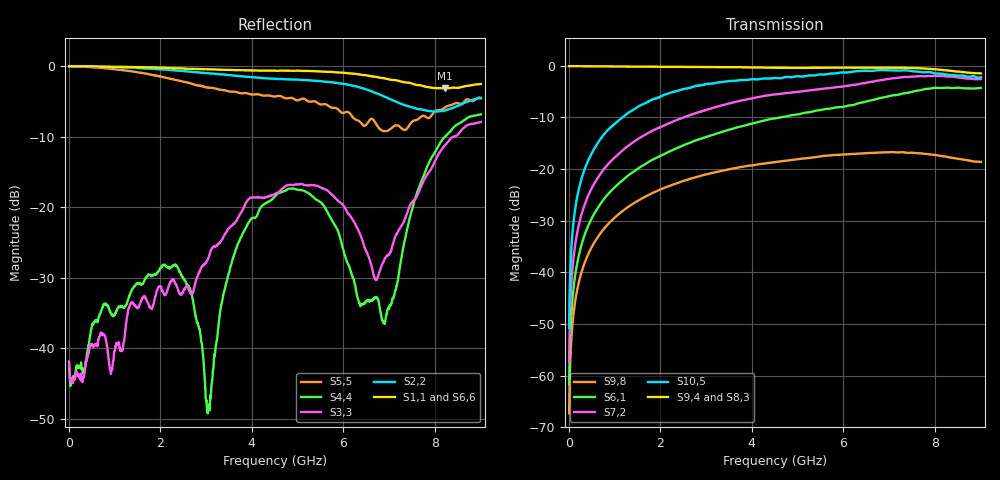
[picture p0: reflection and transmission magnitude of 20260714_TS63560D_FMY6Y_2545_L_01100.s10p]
# GHz S DB R 50
! CMT, SN0916, 25263762, 26.7.0
! Date: 15.07.2026 13:39:32
! Data: Format
! Freq S1.1:dB/Ang S1.2:dB/Ang S1.3:dB/Ang S1.4:dB/Ang S1.5:dB/Ang S1.6:dB/Ang S1.7:dB/Ang S1.8:dB/Ang S1.9:dB/Ang S1.10:dB/Ang
!  S2.1:dB/Ang S2.2:dB/Ang S2.3:dB/Ang S2.4:dB/Ang S2.5:dB/Ang S2.6:dB/Ang S2.7:dB/Ang S2.8:dB/Ang S2.9:dB/Ang S2.10:dB/Ang
!  S3.1:dB/Ang S3.2:dB/Ang S3.3:dB/Ang S3.4:dB/Ang S3.5:dB/Ang S3.6:dB/Ang S3.7:dB/Ang S3.8:dB/Ang S3.9:dB/Ang S3.10:dB/Ang
!  S4.1:dB/Ang S4.2:dB/Ang S4.3:dB/Ang S4.4:dB/Ang S4.5:dB/Ang S4.6:dB/Ang S4.7:dB/Ang S4.8:dB/Ang S4.9:dB/Ang S4.10:dB/Ang
!  S5.1:dB/Ang S5.2:dB/Ang S5.3:dB/Ang S5.4:dB/Ang S5.5:dB/Ang S5.6:dB/Ang S5.7:dB/Ang S5.8:dB/Ang S5.9:dB/Ang S5.10:dB/Ang
!  S6.1:dB/Ang S6.2:dB/Ang S6.3:dB/Ang S6.4:dB/Ang S6.5:dB/Ang S6.6:dB/Ang S6.7:dB/Ang S6.8:dB/Ang S6.9:dB/Ang S6.10:dB/Ang
!  S7.1:dB/Ang S7.2:dB/Ang S7.3:dB/Ang S7.4:dB/Ang S7.5:dB/Ang S7.6:dB/Ang S7.7:dB/Ang S7.8:dB/Ang S7.9:dB/Ang S7.10:dB/Ang
!  S8.1:dB/Ang S8.2:dB/Ang S8.3:dB/Ang S8.4:dB/Ang S8.5:dB/Ang S8.6:dB/Ang S8.7:dB/Ang S8.8:dB/Ang S8.9:dB/Ang S8.10:dB/Ang
!  S9.1:dB/Ang S9.2:dB/Ang S9.3:dB/Ang S9.4:dB/Ang S9.5:dB/Ang S9.6:dB/Ang S9.7:dB/Ang S9.8:dB/Ang S9.9:dB/Ang S9.10:dB/Ang
!  S10.1:dB/Ang S10.2:dB/Ang S10.3:dB/Ang S10.4:dB/Ang S10.5:dB/Ang S10.6:dB/Ang S10.7:dB/Ang S10.8:dB/Ang S10.9:dB/Ang S10.10:dB/Ang
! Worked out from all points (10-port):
!   2001 points, 10 MHz to 9 GHz, reference 50 ohm
!   strongest paths, dB at 10 MHz, 2.257 GHz, 4.505 GHz, 6.753 GHz, 9 GHz:
!     S9,4: -0.1, -0.2, -0.4, -0.4, -1.5
!     S8,3: -0.1, -0.2, -0.4, -0.4, -1.3
!     S10,5: -50.8, -5.1, -2.4, -0.8, -2.2
!     S7,2: -57.4, -10.9, -5.6, -2.9, -2.6
!     S6,1: -61.7, -16.4, -10.2, -6.3, -4.3
!     S9,8: -67.3, -23.1, -18.7, -16.8, -18.6
!   lowest |S11| = -3.2 dB at 8.209 GHz (marker M1), VSWR 5.56, Z = 11.1 - j23.6 ohm
!   |S11| at or under -10 dB: nowhere
